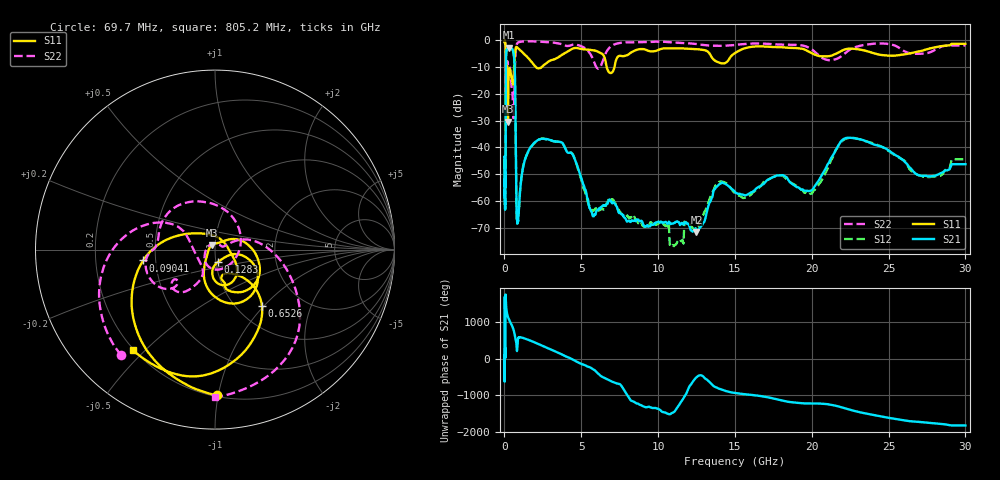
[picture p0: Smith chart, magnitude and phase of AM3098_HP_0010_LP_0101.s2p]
! Date/Time: Thu, Feb 28, 2019 8:32 AM
! Network Analyzer: Agilent Technologies E8364B Rev: A.07.50.67
! Sweep from 0.010 to 30.000 GHz, 1601 Points, Sweep Type: LOG
! Power Supply: 5.023 V, 0.002 A
# Hz S DB R 50
!freq MagS11 AngS11 MagS21 AngS21 MagS12 AngS12 MagS22 AngS22
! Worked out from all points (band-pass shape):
!   1601 points, 10 MHz to 30 GHz, reference 50 ohm
!   highest |S21| = -3.07 dB at 266.5 MHz (marker M1); lowest = -71.3 dB at 12.5 GHz (marker M2)
!   |S21| within 3 dB of the highest: 106.2 MHz to 618.7 MHz (512.5 MHz wide, 141 % of centre)
!   lowest |S11| = -30.4 dB at 227 MHz (marker M3), VSWR 1.06, Z = 48.1 + j2.23 ohm
!   |S11| at or under -10 dB: 175.9 MHz to 632 MHz (456.1 MHz wide, 113 % of centre); 2.02 GHz to 2.458 GHz (438.5 MHz wide, 19.6 % of centre); 6.644 GHz to 7.166 GHz (522 MHz wide, 7.56 % of centre)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
!   |S22| runs from -29.1 to -0.5 dB; largest |S21 - S12| = 0.013
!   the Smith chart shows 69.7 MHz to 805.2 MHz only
!   S11 on the Smith chart (normalised r, x): 69.7 MHz: 0.21, -0.99; 90.41 MHz: 0.43, -0.06; 128.3 MHz: 1.02, -0.14; 652.6 MHz: 1.29, -0.98; 805.2 MHz: 0.20, -0.46
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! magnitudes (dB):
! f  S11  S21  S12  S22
! 10 MHz  -0.3  -43.3  -44.2  -0.5
! 38.04 MHz  -0.5  -59.5  -61.3  -0.9
! 69.7 MHz  -1.8  -51.9  -53.3  -2.1
! 90.41 MHz  -7.9  -19.6  -19.6  -9.3
! 99.92 MHz  -23.8  -8.0  -8.0  -17.3
! 128.3 MHz  -22.9  -4.1  -4.1  -11.0
! 144.7 MHz  -13.7  -3.7  -3.6  -10.3
! 185.8 MHz  -11.3  -3.5  -3.5  -8.1
! 227 MHz  -30.4  -3.2  -3.1  -9.6
! 266.5 MHz  -14.5  -3.1  -3.0  -9.8
! 550.5 MHz  -16.7  -4.1  -4.1  -24.8
! 652.6 MHz  -7.7  -8.7  -8.7  -17.5
! 805.2 MHz  -2.8  -66.3  -66.1  -1.7
! 2.084 GHz  -10.4  -37.6  -37.6  -0.7
! 3.742 GHz  -5.7  -38.2  -38.2  -1.7
! 5.697 GHz  -3.9  -64.1  -63.2  -6.5
! 7.926 GHz  -5.9  -66.9  -64.9  -1.0
! 12.5 GHz  -3.5  -71.3  -69.5  -1.7
! 14.16 GHz  -8.8  -53.0  -52.7  -2.3
! 20 GHz  -5.0  -55.9  -57.1  -3.6
! 22.56 GHz  -3.4  -36.4  -36.5  -3.5
! 30 GHz  -1.6  -46.2  -44.4  -2.2
